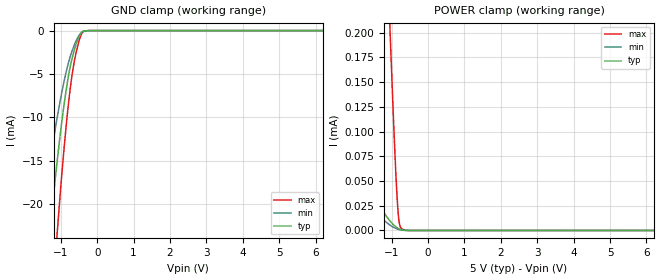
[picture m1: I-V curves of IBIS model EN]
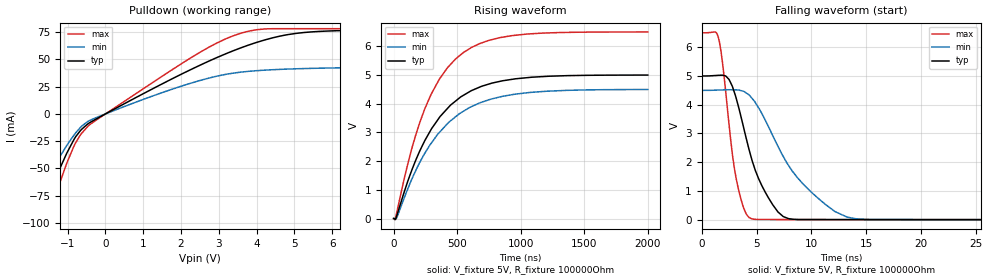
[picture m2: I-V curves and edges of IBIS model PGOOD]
|Texas Instruments Incorporated
|3.3V/5-V Input, 6-A D-CAP+ Mode Synchronous Step-Down, Integrated FET Converter
| Marketing part#   Digital Voltage Range   Package-type   #pins
| TPS531317   4.5-6.5V   RGB   20
[IBIS Ver]   4.1
[File name]   tps51317.ibs
[File Rev]   1.0
[Date]   01/22/2013
[Source]
| Texas Instruments Incorporated.
| Analog-eLab Design Center, HPA
| 12500 TI Blvd
| Dallas, TX -75243
| e-mail: elab_scm_ibis@list.ti.com
[Notes]   Revision History:
| Rev 1.0: 01/22/2013
| - Initial version of the model
| - Model generated from spice simulations
| - C_comp although listed in numerical order of value are
|   obtained from varying PVT conditions. For PVT conditions for
|   each specific value refer the buffer description under
|   respective [Model]. IBIS model user is responsible for using
|   appropriate C_comp to simulate for Signal Integrity.
[Disclaimer]
| This model is designed as an aid for customers of Texas Instruments.
| TI and its licensors and suppliers make no warranties, either expressed
| or implied, with respect to this  model, including the warranties of
| merchantability or fitness for a particular purpose. The model is
| provided solely on an "as is" basis. The entire risk as to its quality
| and performance is with the customer.
[Copyright]
 (C) Copyright 2013 Texas Instruments Incorporated.All rights reserved.
|   TPS51317
[Component]   TPS51317
[Manufacturer]   TI
[Package]   | 20 pin RGP
| variable   typ   min   max
R_pkg   0.05   0.04   0.06
L_pkg   1nH   0.8nH   1.2nH
C_pkg   0.2pF   0.16pF   0.24pF
[Pin]  signal_name   model_name   R_pin   L_pin   C_pin
1   PGND   GND   NA   NA   NA
2   PGND   GND   NA   NA   NA
3   PGND   GND   NA   NA   NA
4   VIN   NC   NA   NA   NA
5   VIN   NC   NA   NA   NA
6   GND   GND   NA   NA   NA
7   VREF   NC   NA   NA   NA
8   COMP   NC   NA   NA   NA
9   REFIN   NC   NA   NA   NA
10   VOUT   NC   NA   NA   NA
11   SW   NC   NA   NA   NA
12   SW   NC   NA   NA   NA
13   SW   NC   NA   NA   NA
14   SW   NC   NA   NA   NA
15   SW   NC   NA   NA   NA
16   BST   NC   NA   NA   NA
17   EN   EN   NA   NA   NA
18   MODE   NC   NA   NA   NA
19   PGOOD   PGOOD   NA   NA   NA
20   V5IN   POWER   NA   NA   NA
| Models and submodels in the file (2): EN (Input), PGOOD (Open_drain)
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|   Model
[Model]   EN
Model_type   Input
Vinl = 0.5
Vinh = 2
|   typ   min   max
C_comp   1.0102pF   0.9413pF   1.1626pF
[Voltage Range]   5   4.5   6.5
[Temperature Range]   27   125   -40
[Power Clamp Reference]   5   4.5   6.5
[GND Clamp Reference]   -0   -0   -0
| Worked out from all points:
|   GND clamp passes 1 mA (typ) near -0.53 V on its own axis
[GND Clamp]
|   Voltage   I(typ)   I(min)   I(max)
-5V       -249.5mA   -179.1mA   -315.5mA
-1.565V   -35.75mA   -23.43mA   -52.52mA
-1.475V   -31.33mA   -20.53mA   -46.48mA
-1.25V    -21.08mA   -13.9mA    -32.12mA
-1.115V   -15.6mA    -10.38mA   -24.18mA
-1.04V    -12.82mA   -8.603mA   -20.06mA
-890mV    -7.912mA   -5.449mA   -12.62mA
-785mV    -5.111mA   -3.625mA   -8.247mA
-695mV    -3.283mA   -2.395mA   -5.211mA
-515mV    -802.2uA   -665.9uA   -1.423mA
-380mV    -60.12uA   -96.16uA   -101.5uA
9.985V    0A         0A         0A
[POWER Clamp]
|   Voltage   I(typ)   I(min)   I(max)
-5V       2.324mA    2.387mA    4.206mA
-2.585V   398.7uA    298.9uA    1.76mA
-2.45V    295.9uA    194.2uA    1.624mA
-2.33V    207uA      110.3uA    1.503mA
-2.18V    104.3uA    43.37uA    1.352mA
-2.015V   38.48uA    33.88uA    1.186mA
-1.07V    10.8uA     6.147uA    228.7uA
-1.04V    9.437uA    5.363uA    199uA
-845mV    2.623uA    1.544uA    30.57uA
-770mV    1.184uA    753.6nA    4.519uA
-620mV    104.8nA    101.8nA    233.3nA
9.985V    0A         0A         0A
|   Model
[Model]   PGOOD
Model_type   Open_drain
Polarity   Non-Inverting
Vmeas = 2.5
Vref = 5
Cref = 1pF
Rref = 100000
|   typ   min   max
C_comp   1.4582pF   1.3278pF   1.5232pF
[Voltage Range]   5   4.5   6.5
[Temperature Range]   27   125   -40
[Pullup Reference]   5   4.5   6.5
[Pulldown Reference]   -0   -0   -0
[Power Clamp Reference]   5   4.5   6.5
[GND Clamp Reference]   -0   -0   -0
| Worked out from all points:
|   slope of the pulldown table from 0 to 0.75 V, typ, clamps not added: 53.7 ohm
|   falling waveform, V_fixture 5V, R_fixture 100000Ohm: 20-80 % time 2.43ns typ, 4.55ns min, 1.24ns max; typ from 5 V to 0.003 V
|   rising waveform, V_fixture 5V, R_fixture 100000Ohm: 20-80 % time 372ns typ, 403ns min, 336ns max; typ from 0.003 V to 5 V
[Pulldown]
|   Voltage   I(typ)   I(min)   I(max)
-5V       -402.2mA   -361.6mA   -457.8mA
-2.165V   -135.7mA   -105mA     -168.8mA
-1.76V    -97.46mA   -74.8mA    -122.4mA
-1.595V   -82.59mA   -63.45mA   -104mA
-1.25V    -53.33mA   -41.67mA   -67.24mA
-830mV    -23.24mA   -19.23mA   -29.2mA
-470mV    -9.248mA   -6.993mA   -11.53mA
2.11V     38.16mA    26.58mA    48.24mA
3.37V     57.77mA    37.35mA    71.51mA
4V        65.6mA     39.65mA    77.22mA
5.26V     74.69mA    41.6mA     78.17mA
9.985V    79.72mA    46.06mA    78.17mA
[Ramp]
R_load = 100000
|   typ   min   max
dV/dt_r   2.9981/3.72511e-07   2.69635/4.02685e-07   3.89856/3.35937e-07
dV/dt_f   2.99841/2.42675e-09   2.69729/4.54888e-09   3.89834/1.2381e-09
[Falling Waveform]
V_fixture = 5V
V_fixture_min = 4.5V
V_fixture_max = 6.5V
R_fixture = 100000Ohm
C_fixture = 0F
|   Time   V(typ)   V(min)   V(max)
0s        5V         4.499V     6.5V
1.498ns   5.022V     4.509V     6.378V
2.5ns     4.877V     4.521V     3.303V
3.292ns   4.024V     4.514V     1.169V
4.065ns   2.828V     4.407V     195.1mV
5.368ns   1.281V     3.776V     10.28mV
7.442ns   109mV      2.197V     7.194mV
9.921ns   7.682mV    984.9mV    5.535mV
15.6ns    4.694mV    9.362mV    3.833mV
2us       2.6mV      3.228mV    2.743mV
[Rising Waveform]
V_fixture = 5V
V_fixture_min = 4.5V
V_fixture_max = 6.5V
R_fixture = 100000Ohm
C_fixture = 0F
|   Time   V(typ)   V(min)   V(max)
0s        2.6mV      3.228mV    2.743mV
13.21ns   -31.87mV   -3.226mV   -15.18mV
26.73ns   122.2mV    50.04mV    247.2mV
134.4ns   1.58V      1.28V      2.291V
245.2ns   2.712V     2.271V     3.819V
359.3ns   3.513V     2.996V     4.851V
550.2ns   4.296V     3.741V     5.786V
677.4ns   4.58V      4.029V     6.095V
930.2ns   4.849V     4.315V     6.372V
2us       4.999V     4.497V     6.5V
